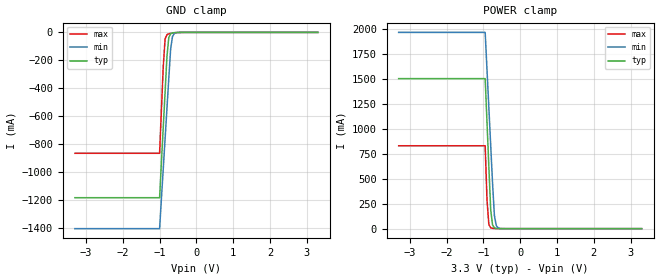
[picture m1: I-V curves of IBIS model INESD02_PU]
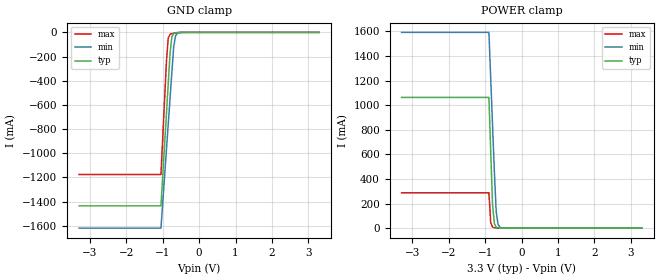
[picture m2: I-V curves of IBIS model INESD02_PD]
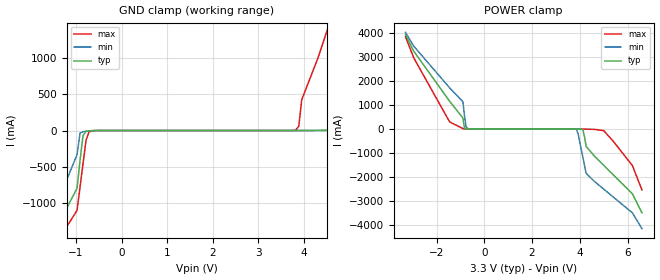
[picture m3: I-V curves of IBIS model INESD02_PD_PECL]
|   This file is an IBIS representation of the   |
|   Integrated Device Technology, Inc.   |
|   ICS85102I   |
|   LOW SKEW, 1-TO-2, DIFFERENTIAL/LVCMOS-TO-0.7V HCSL FANOUT BUFFER   |
[IBIS Ver]   4.1
[File name]   85102i_3v3.ibs
[File Rev]   4.0
[Date]   7 Aug 2009 | Last modified
|   May 07 2007 | Generated
[Source]   Originated at Integrated Device Technology, Inc.
[Disclaimer]
IDT hereby grants the user of this IBIS model a non-exclusive,
nontransferable license to use this IBIS model under the following terms.
Before using this IBIS model, the user should read this license.
If the user does not accept these terms,  the IBIS model should be
returned to IDT within 30 days.
   The user is granted this license only to use the IBIS model and
is not granted rights to sell, load, rent, lease or license the IBIS
model in whole or in part, or in modified form to anyone other than
user. User may modify the IBIS model to suit its specific
applications but rights to derivative works and such modifications
shall belong to IDT.
   This IBIS model is provided on an "AS IS" basis and IDT makes
absolutely no warranty with respect to the information contained
herein. IDT DISCLAIMS AND CUSTOMER WAIVES ALL WARRANTIES, EXPRESS
OR IMPLIED, INCLUDING WARRANTIES OF MERCHANTABILITY OR FITNESS FOR
A PARTICULAR PURPOSE. The entire risk as to quality and performance
is with the Customer. ACCORDINGLY, IN NO EVENT SHALL THE COMPANY BE
LIABLE FOR ANY DAMAGES, WHETHER IN CONTRACT OR TORT,INCLUDING ANY
LOST PROFITS OR OTHER INCIDENTAL, CONSEQUENTIAL, EXEMPLARY, OR
PUNITIVE DAMAGES ARISING OUT OF THE USE OR APPLICATION OF THE IBIS
model provided in this package. Further, IDT reserves the right to
make changes without notice to any product herein to improve
reliability, function, or design. IDT does not convey any license
under patent rights or any other intellectual property rights,
including those of third parties.
   IDT is not obligated to provide maintenance or support
for the licensed IBIS model.
[Copyright]   Copyright 2006 by Integrated Device Technology, Inc.
[Component]   ICS85102AGI
[Manufacturer] Integrated Device Technology, Inc.
[Package]
| TSSOP16   typ   min   max
R_pkg   58.65m   52.5m   64.8m
L_pkg   1.902nH   1.443nH   2.361nH
C_pkg   0.315pF   0.254pF   0.375pF
[Pin] signal_name   model_name   R_pin   L_pin   C_pin
1   CLK_EN   INESD02_PU   64.8m   2.361n   0.375p
2   CLK_SEL   INESD02_PD   60.7m   2.054n   0.335p
3   CLK0   INESD02_PD_PECL   56.6m   1.749n   0.294p
4   nCLK0   INESD02_PD_PU   52.5m   1.443n   0.254p
5   CLK1   INESD02_PD_PECL   52.5m   1.443n   0.254p
6   nc   NC   56.6m   1.749n   0.294p
7   nc   NC   60.7m   2.054n   0.335p
8   IREF   NC   64.8m   2.361n   0.375p
9   VDD   POWER   64.8m   2.361n   0.375p
10  VDD   POWER   60.7m   2.054n   0.335p
11  nQ1   DCMOUT01_ISO2_OP   56.6m   1.749n   0.294p
12  Q1   DCMOUT01_ISO2_OP   52.5m   1.443n   0.254p
13  nQ0   DCMOUT01_ISO2_OP   52.5m   1.443n   0.254p
14  Q0   DCMOUT01_ISO2_OP   56.6m   1.749n   0.294p
15  VDD   POWER   60.7m   2.054n   0.335p
16  GND   GND   64.8m   2.361n   0.375p
[Diff Pin]   inv_pin  vdiff tdelay_typ tdelay_min  tdelay_max
 3   4   0.15   0   0   0
12   11   NA   0   0   0
14   13   NA   0   0   0
| Models and submodels in the file (5): INESD02_PU (Input), INESD02_PD (Input), INESD02_PD_PECL (Input), INESD02_PD_PU (Input), DCMOUT01_ISO2_OP (Open_source)
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[Model]   INESD02_PU
Model_type   Input
Polarity   Non-Inverting
Vinl = 0.80V
Vinh = 2.0V
|   typ   min   max
C_comp   2pF   1.5pF   2.5pF
|   typ   min   max
[Voltage range]  3.3V   3.15V   3.45V
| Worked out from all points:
|   GND clamp passes 1 mA (typ) near -0.56 V on its own axis
|   POWER clamp passes 1 mA (typ) near -0.61 V on its own axis
[GND_clamp]
|Voltage   I(typ)   I(min)   I(max)
-3.3V     -1.184A    -1.405A    -865.6mA
-1V       -1.184A    -1.405A    -865.6mA
-900mV    -678.5mA   -975.1mA   -244.1mA
-850mV    -426.2mA   -760.2mA   -46.92mA
-800mV    -174mA     -545.4mA   -16.17mA
-750mV    -37.03mA   -330.8mA   -9.981mA
-700mV    -9.767mA   -120.3mA   -7.122mA
-650mV    -3.616mA   -29.78mA   -4.922mA
-600mV    -1.7mA     -7.594mA   -3.115mA
-400mV    -123.9uA   -126uA     -173.9uA
3.3V      1.866nA    3.949uA    0A
[POWER_clamp]
|Voltage   I(typ)   I(min)   I(max)
-3.3V     1.506A     1.97A      832.1mA
-950mV    1.506A     1.97A      832.1mA
-900mV    1.063A     1.592A     287.2mA
-850mV    620.4mA    1.215A     41.77mA
-800mV    191.5mA    837.4mA    8.692mA
-750mV    37.69mA    460.1mA    3.262mA
-700mV    8.032mA    133.8mA    1.662mA
-650mV    2.005mA    32.58mA    840.1uA
-600mV    607uA      8.009mA    378.6uA
-450mV    33.11uA    139.8uA    23.88uA
3.3V      -71.13uA   -77.46uA   -62.11uA
[Model]   INESD02_PD
Model_type   Input
Polarity   Non-Inverting
Vinl = 0.80V
Vinh = 2.0V
|   typ   min   max
C_comp   2pF   1.5pF   2.5pF
|   typ   min   max
[Voltage range]  3.3V   3.15V   3.45V
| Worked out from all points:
|   GND clamp passes 1 mA (typ) near -0.56 V on its own axis
|   POWER clamp passes 1 mA (typ) near -0.61 V on its own axis
[GND_clamp]
|Voltage   I(typ)   I(min)   I(max)
-3.3V     -1.436A    -1.62A     -1.176A
-1.05V    -1.436A    -1.62A     -1.176A
-900mV    -678.5mA   -975.1mA   -244mA
-850mV    -426.1mA   -760.1mA   -46.85mA
-800mV    -173.9mA   -545.4mA   -16.11mA
-750mV    -36.96mA   -330.7mA   -9.916mA
-700mV    -9.696mA   -120.2mA   -7.056mA
-650mV    -3.545mA   -29.7mA    -4.857mA
-600mV    -1.629mA   -7.52mA    -3.049mA
-400mV    -52.81uA   -52.52uA   -108.7uA
3.3V      71.13uA    77.43uA    62.11uA
[POWER_clamp]
|Voltage   I(typ)   I(min)   I(max)
-3.3V     1.063A     1.593A     287.3mA
-900mV    1.063A     1.593A     287.3mA
-850mV    620.5mA    1.215A     41.84mA
-800mV    191.6mA    837.5mA    8.757mA
-750mV    37.76mA    460.2mA    3.328mA
-700mV    8.104mA    133.8mA    1.728mA
-650mV    2.076mA    32.66mA    905.3uA
-600mV    678.1uA    8.083mA    443.8uA
-450mV    104.2uA    213.3uA    89.09uA
3.3V      -3.041nA   -3.986uA   0A
[Model]   INESD02_PD_PECL
Model_type  Input
Polarity   Non-Inverting
Vinl = 0.8V
Vinh = 2.0V
|   typ   min   max
C_comp   2pF   1.5pF   2.5pF
|   typ   min   max
[Voltage range]  3.3V   3.15V   3.45V
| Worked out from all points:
|   GND clamp passes 1 mA (typ) near -0.59 V on its own axis
|   POWER clamp passes 1 mA (typ) near -0.70 V on its own axis
[GND_clamp]
-3.3V     -3.894A    -4.294A    -3.674A
-1.6V     -1.569A    -1.322A    -1.74A
-974.8mV  -794.1mA   -331.5mA   -1.096A
-843.4mV  -68.33mA   -15.34mA   -452.9mA
-646.5mV  -1.912mA   -4.151mA   -2.665mA
3.818V    89.38uA    70.49uA    7.198mA
3.95V     342.2uA    75.94uA    423.8mA
4.6V      7.437mA    165.5uA    1.553A
4.9V      78.32mA    440.9uA    2.118A
5.5V      1.293A     2.769mA    3.249A
6.25V     2.651A     112.4mA    4.38A
6.6V      3.331A     896.1mA    4.946A
[POWER_clamp]
-3.3V     3.923A     4.017A     3.838A
-2.95V    3.23A      3.44A      2.951A
-1.45V    1.149A     1.709A     289.6mA
-896.9mV  456.5mA    1.133A     15.4mA
-762.9mV  4.223mA    91.07mA    1.486mA
-695.9mV  792.2uA    10.73mA    555.6uA
3.861V    -556.7uA   -26.14mA   -39.45uA
4.129V    -41.85mA   -1.19A     -4.904mA
4.263V    -724.2mA   -1.847A    -12.04mA
5V        -1.514A    -2.505A    -71.38mA
6.2V      -2.701A    -3.492A    -1.525A
6.6V      -3.492A    -4.151A    -2.536A
